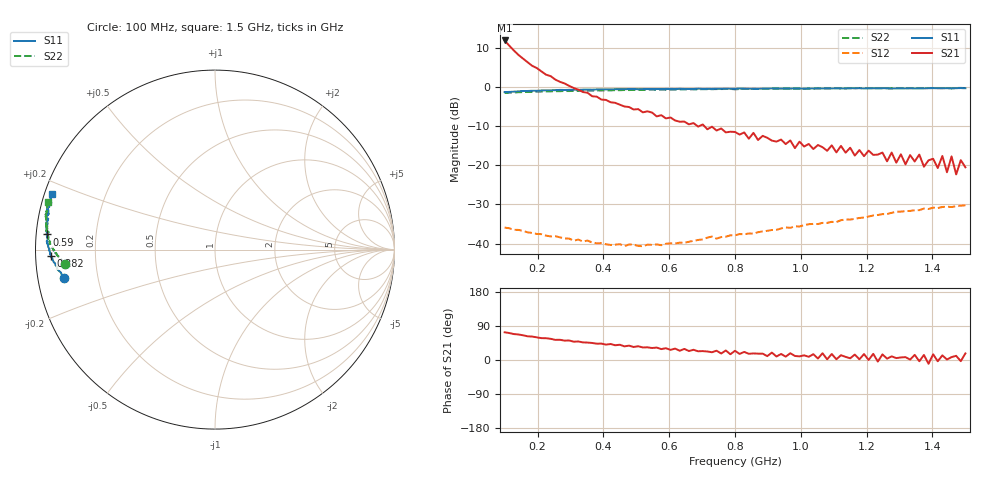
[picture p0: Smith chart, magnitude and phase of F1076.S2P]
!  POLYFET RF DEVICES
!  S PARAMETERS FOR
!  F1076 (Each Side)
!  VDS=28, IDQ=800mA
! Date: Mon Oct 21 18:10:46 1991
! Bias (V mA) : V1=2.5299000  I1=0.0051051  V2=27.993660  I2=702.49320
# MHZ S MA R 50
!  FREQ  S11 MAG  S11 ANG  S21 MAG  S21 ANG  S12 MAG  S12 ANG  S22 MAG  S22 ANG
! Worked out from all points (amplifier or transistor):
!   101 points, 100 MHz to 1.5 GHz, reference 50 ohm
!   highest |S21| = 11.8 dB at 100 MHz (marker M1)
!   |S21| within 3 dB of that: start of sweep to 133.6 MHz
!   unconditionally stable (mu >= 1): 352.6 MHz to 1.146 GHz; 1.237 GHz to 1.327 GHz; 1.401 GHz to 1.477 GHz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
!   at 324 MHz: K = 0.99, MSG = 19.1 dB, |S12| = -39.0 dB
!   at 800 MHz: K = 2.04, MAG = 7.4 dB, |S12| = -37.9 dB
!   at 1.5 GHz: K = 1.28, MAG = 1.6 dB, |S12| = -30.2 dB
!   S11 on the Smith chart (normalised r, x): 100 MHz: 0.08, -0.09; 282 MHz: 0.05, -0.02; 590 MHz: 0.03, +0.04; 1.5 GHz: 0.02, +0.17
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100  0.8579 -169.5  3.91 73.2  0.01604 -6.7  0.8373 -174.4
128  0.8681 -171.6  2.918 68.5  0.01505 -9.3  0.8483 -175.6
170  0.8868 -174.0  2.06 62.5  0.01396 -8.6  0.863 -176.7
226  0.9046 -176.2  1.431 57.5  0.01267 -6.6  0.8735 -177.5
282  0.9132 -177.8  1.107 51.1  0.01165 -5.7  0.8861 -178.6
338  0.9219 -179.5  0.8598 46.4  0.01065 -0.5  0.8916 -179.5
576  0.9363 175.2  0.4354 28.8  0.00956 29.6  0.9246 177.2
590  0.9422 174.8  0.3961 31.2  0.00998 32.4  0.9197 176.9
800  0.9454 171.3  0.2661 24.3  0.0128 48.7  0.931 174.1
1038  0.9521 167.0  0.1611 15.4  0.01788 61.9  0.951 170.6
1262  0.9595 164.3  0.1124 3.6  0.02385 65.4  0.9607 167.1
1276  0.9479 164.0  0.1452 9.6  0.02476 65.9  0.9638 167.2
1290  0.9596 163.8  0.108 5.0  0.02551 65.8  0.9613 166.8
1360  0.9574 162.9  0.1369 -3.3  0.02676 64.1  0.9633 165.9
1374  0.9575 162.6  0.09591 13.3  0.02802 64.1  0.9622 165.8
1416  0.9599 162.3  0.09218 -3.3  0.02845 64.5  0.9662 165.0
1430  0.9589 161.8  0.1315 12.2  0.02938 63.4  0.9656 165.3
1444  0.9607 161.9  0.08144 1.3  0.02964 64.2  0.9689 164.7
1458  0.9528 161.6  0.1297 7.7  0.02932 63.8  0.9643 164.8
1472  0.9618 160.9  0.07643 11.1  0.03012 63.0  0.9689 164.5
1486  0.9654 161.0  0.1161 -3.1  0.0305 63.1  0.9704 164.5
1500  0.9602 161.0  0.09426 17.4  0.03085 63.3  0.9666 164.0
